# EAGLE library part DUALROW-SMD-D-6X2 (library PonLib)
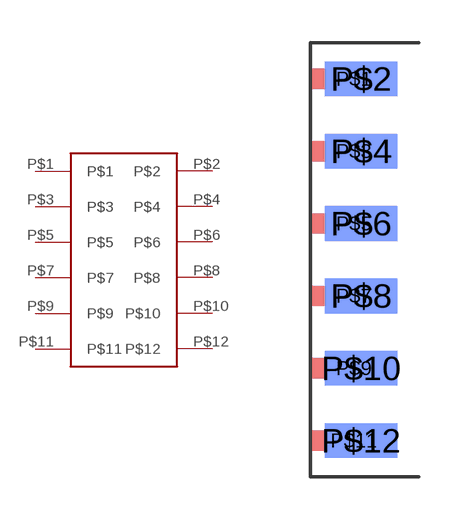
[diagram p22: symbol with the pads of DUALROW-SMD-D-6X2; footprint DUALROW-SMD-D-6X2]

Designator prefix -

## DUALROW-SMD-D-6X2  [DUALROW-SMD-D-6X2]
P$1  P$1
P$2  P$2
P$3  P$3
P$4  P$4
P$5  P$5
P$6  P$6
P$7  P$7
P$8  P$8
P$9  P$9
P$10  P$10
P$11  P$11
P$12  P$12

## Footprint DUALROW-SMD-D-6X2 (pad centres in mm)
smd 3.048 x 0.711: P$1 1.524,6.35; P$3 1.524,3.81; P$5 1.524,1.27; P$7 1.524,-1.27; P$9 1.524,-3.81; P$11 1.524,-6.35
smd 2.54 x 1.219 bottom: P$2 1.778,6.35; P$4 1.778,3.81; P$6 1.778,1.27; P$8 1.778,-1.27; P$10 1.778,-3.81; P$12 1.778,-6.35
